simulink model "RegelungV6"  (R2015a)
settings: Solver=ode45  StartTime=0.0  StopTime=5  MaxStep=1e-2  MinStep=1e-3  RelTol=1e-3
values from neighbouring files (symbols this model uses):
  iFeedbackOn = 1    [Versuch6.m]
  iForceInput = 0    [Versuch6.m]
  Mges = stPendel.mPendel + stPendel.mSchlitten    [Versuch6.m]
  mK = zeros(length(vT), n)    [berechneK.m]
  stPendel = block.DialogPrm(1).Data    [systemPendel_V3.m]    (also in systemPendel_V5.m; Versuch6.m = ladePendel(); Versuch3.m = ladePendel(); simGUI.m = ladePendel())
  stTraj = l.caTraj{2}    [Versuch6.m]    (also in Versuch5_A_Berechnung.m = caTraj{1}; Versuch5_C_Simulation_mit_Simulink.m = berechneTrajektorie(stPendel, 1.2))
  T_Motor = 0.01    [Versuch6.m]
  x0 = block.DialogPrm(2).Data    [systemPendel_V3.m]    (also in systemPendel_V5.m; Versuch6.m = [0 0 0 0].'; Versuch3.m = [0.5 0 1*AP 0]; simGUI.m = [x1_0 x2_0 x3_0 x4_0])
undefined symbols (not defined in the file or in its folder): interp1, vTK

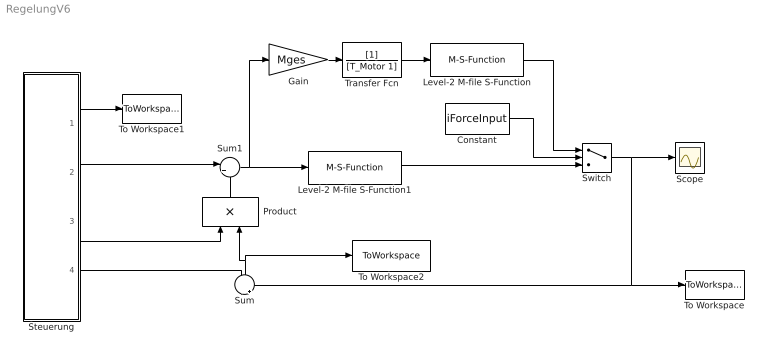
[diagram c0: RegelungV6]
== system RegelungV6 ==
  Constant : Constant  Value=iForceInput
  Gain : Gain  Gain=Mges
  Level-2 M-file S-Function : M-S-Function  FunctionName=systemPendel_V3  Parameters=stPendel,x0
  Level-2 M-file S-Function1 : M-S-Function  FunctionName=systemPendel_V5  Parameters=stPendel,x0
  Product : Product  Multiplication=Matrix(*)
  Scope : Scope
  Steuerung : Subsystem
  Sum : Sum  Inputs=-|+
  Sum1 : Sum  Inputs=|+-
  Switch : Switch  Criteria=u2 ~= 0
  To Workspace : ToWorkspace  VariableName=mStates  SampleTime=-1
  To Workspace1 : ToWorkspace  VariableName=vT  SampleTime=-1
  To Workspace2 : ToWorkspace  VariableName=mDeltaStates  SampleTime=-1
  Transfer Fcn : TransferFcn  Denominator=[T_Motor 1]
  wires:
  Steuerung/1(t) -> To Workspace1/1
  Steuerung/4(x*) -> Sum/1
  Sum/1 -> Product/2, To Workspace2/1
  Steuerung/3(K*) -> Product/1
  Steuerung/2(u*) -> Sum1/1
  Sum1/1 -> Level-2 M-file S-Function1/1, Gain/1
  Product/1 -> Sum1/2
  Gain/1 -> Transfer Fcn/1
  Transfer Fcn/1 -> Level-2 M-file S-Function/1
  Level-2 M-file S-Function/1 -> Switch/1
  Level-2 M-file S-Function1/1 -> Switch/3
  Switch/1 -> Scope/1, To Workspace/1, Sum/2
  Constant/1 -> Switch/2

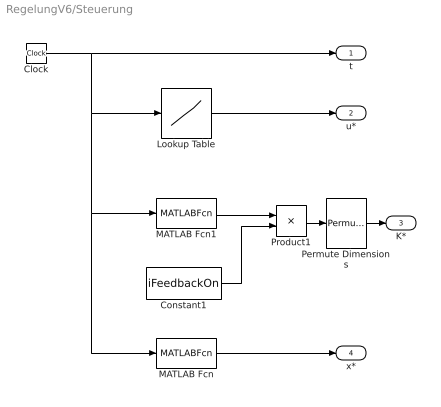
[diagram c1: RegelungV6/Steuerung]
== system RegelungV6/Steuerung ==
  Clock : Clock
  Constant1 : Constant  Value=iFeedbackOn
  Lookup Table : Lookup  InputValues=stTraj.vT  Table=stTraj.vU  LookUpMeth=Interpolation-Use End Values
  MATLAB Fcn : MATLABFcn  MATLABFcn=interp1(stTraj.vT, stTraj.mX', u, 'nearest', 'extrap')'  OutputDimensions=4
  MATLAB Fcn1 : MATLABFcn  MATLABFcn=interp1(vTK, mK, u, 'nearest', 'extrap')  OutputDimensions=4
  Permute Dimensions : PermuteDimensions
  Product1 : Product
  t : Outport
  u* : Outport  Port=2
  K* : Outport  Port=3
  x* : Outport  Port=4
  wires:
  Lookup Table/1 -> u*/1
  Clock/1 -> t/1, Lookup Table/1, MATLAB Fcn1/1, MATLAB Fcn/1
  MATLAB Fcn/1 -> x*/1
  MATLAB Fcn1/1 -> Product1/1
  Product1/1 -> Permute Dimensions/1
  Constant1/1 -> Product1/2
  Permute Dimensions/1 -> K*/1
